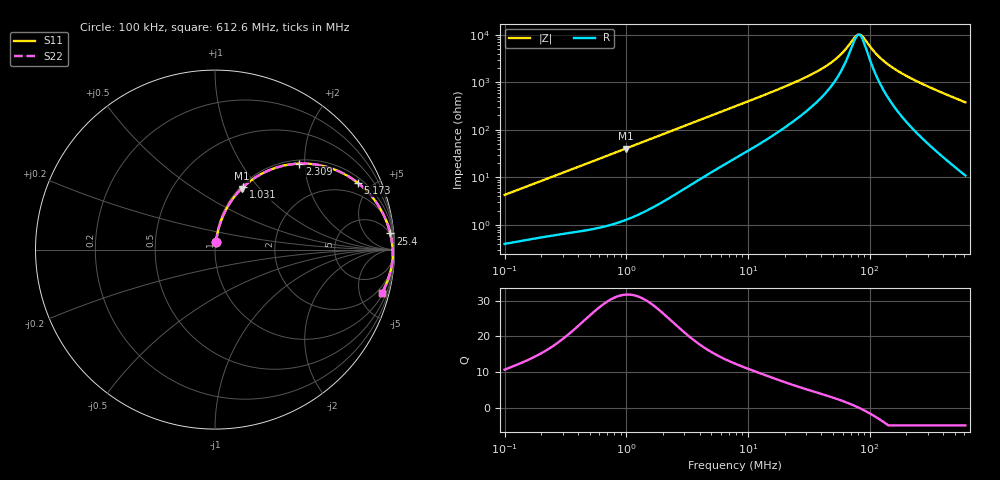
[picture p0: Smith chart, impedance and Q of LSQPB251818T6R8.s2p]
! LSQPB251818T6R8  S-PARAMETER MODEL  ( General Type )
! Model Generated by TAIYO YUDEN Corporation (http://www.ty-top.com)
! Version 2.0
! TAIYO YUDEN Control No. 100810NG19SB-FKC
! Copyright(c) 2009 TAIYO YUDEN CO.,LTD. All Rights Reserved.
! Product Description (link to TY-COMPAS)
! https://ds.yuden.co.jp/TYCOMPAS/or/detail?pn=LSQPB251818T6R8M&u=M
! Products Name : Inductors
! Characteristics :
!  Inductance : 6.8 uH , SRF(min) : 45 MHz , DC Resistance(max) : 0.364 Ohm
!  Rated Current : Saturation :1050 mA , Temp Rise : 680 mA (40 degC)
!  Case Size : 2.5 x 1.8 / 0.098 x 0.071 [mm/inch] , Thickness : 1.8 / 0.071 [mm/inch]
!  (Conditions: Temperature = 25 degC , DC Bias Current/Voltage = 0A / 0V)
! External Node Assignments :
!  1  o---GGG---o  2
! GND o---------o GND
! Frequency Range : 0.1MHz  -  612.621916MHz  [ 402 STEP ]
# MHz S RI R 50
! Freq[MHz].  S11 Real  S11 Imag  S21 Real  S21 Imag  S12 Real  S12 Imag  S22 Real  S22 Imag
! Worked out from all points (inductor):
!   401 points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, 100 kHz to 612.6 MHz, reference 50 ohm
!   read as one part in series: L = 6.75 uH near 104.5 kHz
!   highest Q = 31.7 at 986.6 kHz (marker M1), where L = 6.51 uH
!   self-resonance near 80.66 MHz
!   S11 on the Smith chart (normalised r, x): 100 kHz: 1.01, +0.09; 1.031 MHz: 1.03, +0.84; 2.309 MHz: 1.08, +1.88; 5.173 MHz: 1.27, +4.14; 25.4 MHz: 4, +21; 612.6 MHz: 1.22, -7.55
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0.1  0.00578 0.0423  0.9942 -0.0423  0.9942 -0.0423  0.00578 0.0423
0.224035  0.0142 0.0916  0.9858 -0.0916  0.9858 -0.0916  0.0142 0.0916
0.430878  0.0373 0.1696  0.9627 -0.1696  0.9627 -0.1696  0.0373 0.1696
0.986593  0.148 0.3397  0.852 -0.3397  0.852 -0.3397  0.148 0.3397
1.030562  0.1587 0.35  0.8413 -0.35  0.8413 -0.35  0.1587 0.35
1.856562  0.3688 0.4646  0.6312 -0.4646  0.6312 -0.4646  0.3688 0.4646
2.308816  0.4699 0.4792  0.5301 -0.4792  0.5301 -0.4792  0.4699 0.4792
3.27248  0.6307 0.4583  0.3693 -0.4583  0.3693 -0.4583  0.6307 0.4583
5.172549  0.7961 0.3716  0.2039 -0.3716  0.2039 -0.3716  0.7961 0.3716
7.827017  0.8878 0.2777  0.1122 -0.2777  0.1122 -0.2777  0.8878 0.2777
25.40196  0.9762 0.0903  0.0238 -0.0903  0.0238 -0.0903  0.9762 0.0903
33.72493  0.9819 0.0638  0.0181 -0.0638  0.0181 -0.0638  0.9819 0.0638
43.80935  0.9855 0.0429  0.0145 -0.0429  0.0145 -0.0429  0.9855 0.0429
53.30631  0.9875 0.0287  0.0125 -0.0287  0.0125 -0.0287  0.9875 0.0287
62.09469  0.9887 0.0182  0.0113 -0.0182  0.0113 -0.0182  0.9887 0.0182
75.55554  0.9899 0.00491  0.0101 -0.00491  0.0101 -0.00491  0.9899 0.00491
80.66224  0.9902 0.000476  0.00985 -0.000476  0.00985 -0.000476  0.9902 0.000476
88.01206  0.9904 -0.00548  0.00957 0.00548  0.00957 0.00548  0.9904 -0.00548
114.3294  0.9906 -0.024  0.00937 0.024  0.00937 0.024  0.9906 -0.024
145.3134  0.9899 -0.0426  0.0101 0.0426  0.0101 0.0426  0.9899 -0.0426
256.1376  0.9824 -0.0984  0.0176 0.0984  0.0176 0.0984  0.9824 -0.0984
612.6219  0.9284 -0.2437  0.0716 0.2437  0.0716 0.2437  0.9284 -0.2437
